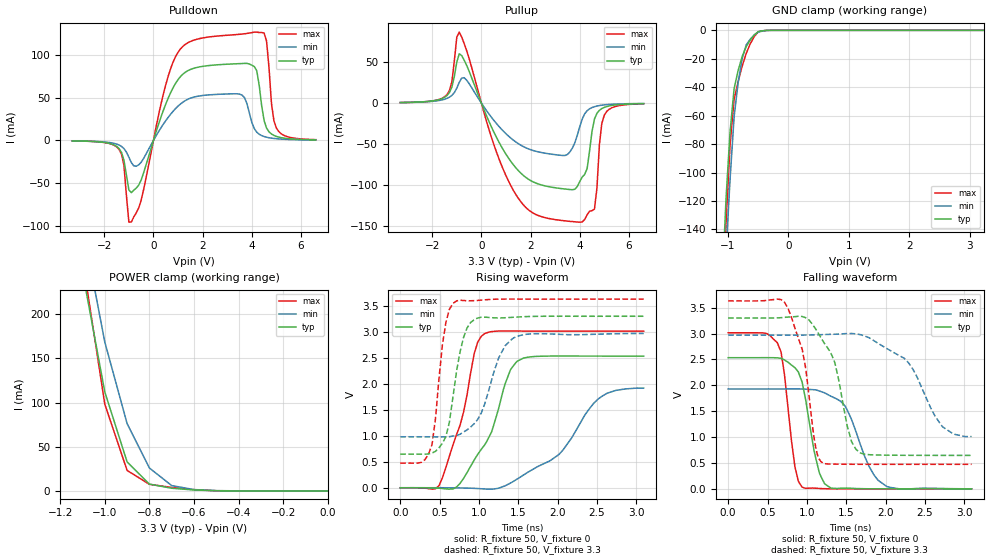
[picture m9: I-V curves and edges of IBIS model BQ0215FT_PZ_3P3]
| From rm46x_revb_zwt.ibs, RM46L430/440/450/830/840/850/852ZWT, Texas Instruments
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|   Model Cell BQ0215FT_PZ_3P3
|BQ0215FT_PZ_3P3
[Model]   BQ0215FT_PZ_3P3
Model_type   I/O
Polarity   Non-Inverting
Enable   Active-Low
Vinl =  1.15
Vinh =  1.55
Cref =  15.0001pF
Rref =  101.0000M
Vref =  0V
Vmeas =  1.65
C_comp   1.2p   1.2p   1.2p
[Model Spec]
Vinl   1.15   1.02   1.28
Vinh   1.55   1.45   1.65
[Temperature Range]   25   155   -40
[Voltage Range]   3.3   2.97   3.63
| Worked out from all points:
|   slope of the pulldown table from 0 to 0.495 V, typ, clamps not added: 11.7 ohm
|   slope of the pullup table from 0 to 0.495 V, typ, clamps not added: 14.3 ohm
|   GND clamp passes 1 mA (typ) near -0.50 V on its own axis
|   POWER clamp passes 1 mA (typ) near -0.59 V on its own axis
|   rising waveform, R_fixture 50, V_fixture 0: 20-80 % time 410ps typ, 692ps min, 296ps max; typ from 0 V to 2.53 V
|   rising waveform, R_fixture 50, V_fixture 3.3: 20-80 % time 174ps typ, 268ps min, 133ps max; typ from 0.647 V to 3.3 V
|   falling waveform, R_fixture 50, V_fixture 0: 20-80 % time 182ps typ, 302ps min, 138ps max; typ from 2.53 V to 0 V
|   falling waveform, R_fixture 50, V_fixture 3.3: 20-80 % time 278ps typ, 461ps min, 209ps max; typ from 3.3 V to 0.646 V
[POWER_clamp]
|   voltage   I(typ)   I(min)   I(max)
-3.3V     4.034A     4.621A     4.844A
-1.1V     248.3mA    300.9mA    262.9mA
-1.067V   202.9mA    256.8mA    208mA
-1.033V   157.5mA    212.7mA    153.2mA
-1V       112.1mA    168.6mA    98.31mA
-900mV    32.88mA    76.22mA    23.22mA
-800mV    7.705mA    25.94mA    7.475mA
-700mV    3.033mA    6.038mA    3.991mA
-600mV    1.087mA    1.528mA    1.425mA
-500mV    187uA      368.9uA    203.4uA
0V        579.1pA    13.17nA    479.4pA
[Pulldown]
|   voltage   I(typ)   I(min)   I(max)
-3.3V     -583.8uA   -509.7uA   -562.9uA
-1.4V     -9.427mA   -5.344mA   -10.39mA
-1.2V     -23.28mA   -9.543mA   -29.38mA
-1V       -58.07mA   -19.65mA   -95.88mA
-900mV    -61.21mA   -25.99mA   -95.59mA
1V        71.34mA    40.23mA    103.4mA
3.5V      90.06mA    54.34mA    124.5mA
4.2V      81.77mA    9.741mA    127mA
4.6V      14.51mA    3.766mA    116.4mA
4.8V      7.515mA    2.688mA    43.16mA
5V        4.703mA    2.013mA    14.54mA
6.6V      667.2uA    491.6uA    918.8uA
[Pullup]
|   voltage   I(typ)   I(min)   I(max)
-3.3V     645.2uA    598.5uA    584.2uA
-1.4V     9.107mA    5.632mA    10.27mA
-900mV    59.97mA    25.19mA    86.39mA
600mV     -40.93mA   -24.45mA   -58.47mA
1.4V      -78.76mA   -47.33mA   -111.2mA
3.4V      -104.6mA   -63.8mA    -143.4mA
4V        -95.69mA   -28.77mA   -145mA
4.3V      -79.78mA   -9.339mA   -136mA
4.6V      -19.38mA   -4.395mA   -129mA
4.8V      -8.841mA   -3.032mA   -50.9mA
5V        -5.243mA   -2.22mA    -14.75mA
6.6V      -699.3uA   -541.6uA   -880.5uA
[GND_clamp]
|   voltage   I(typ)   I(min)   I(max)
-3.3V     -3.232A    -2.867A    -4.906A
-1.1V     -181.4mA   -214mA     -212mA
-1.033V   -118mA     -155.8mA   -134.9mA
-966.7mV  -71.18mA   -104.7mA   -80.42mA
-900mV    -40.99mA   -60.83mA   -48.65mA
-833.3mV  -28.23mA   -36.87mA   -36.01mA
-766.7mV  -18.41mA   -20mA      -25.23mA
-700mV    -11.54mA   -10.23mA   -16.3mA
-566.7mV  -3.309mA   -3.247mA   -4.437mA
-500mV    -880.1uA   -1.256mA   -1.015mA
-300mV    -1.832uA   -15.98uA   -900.8nA
3.233V    553.4pA    4.097uA    367.7pA
[Ramp]
| variable   typ   min   max
dV/dt_f   1.613268/0.2883466n   1.213022/0.4924881n   1.916193/0.2144453n
dV/dt_r   1.537386/0.417794n   1.174541/0.7163023n   1.826409/0.2991251n
R_load = 50
[Rising Waveform]
R_fixture = 50
V_fixture = 0
V_fixture_min = 0
V_fixture_max = 0
|   time   V(typ)   V(min)   V(max)
0s        -1.134uV   -4.139uV   -934.2nV
492ps     -9.176mV   409.8uV    39.5mV
716ps     14.01mV    -2.646mV   1.026V
804ps     179.4mV    -5.212mV   1.456V
940ps     533.9mV    -11.54mV   2.583V
1.072ns   823mV      -23.66mV   2.966V
1.488ns   2.437V     169.9mV    3.015V
2.016ns   2.534V     640.6mV    3.014V
2.516ns   2.533V     1.711V     3.014V
3.092ns   2.533V     1.917V     3.014V
[Rising Waveform]
R_fixture = 50
V_fixture = 3.3
V_fixture_min = 2.97
V_fixture_max = 3.63
|   time   V(typ)   V(min)   V(max)
0s        646.5mV    980.1mV    473.8mV
268ps     646mV      980.2mV    487.6mV
404ps     667.9mV    979.6mV    831.7mV
580ps     985.4mV    979.7mV    3.183V
716ps     2.248V     1.007V     3.596V
892ps     3.177V     1.164V     3.598V
1.028ns   3.281V     1.434V     3.61V
1.248ns   3.267V     2.488V     3.629V
1.444ns   3.281V     2.886V     3.631V
3.092ns   3.3V       2.968V     3.63V
[Falling Waveform]
R_fixture = 50
V_fixture = 0
V_fixture_min = 0
V_fixture_max = 0
|   time   V(typ)   V(min)   V(max)
0s        2.534V     1.93V      3.014V
624ps     2.53V      1.93V      2.825V
716ps     2.49V      1.93V      2.204V
848ps     2.341V     1.931V     428.5mV
940ps     2.06V      1.929V     31.58mV
1.16ns    301.6mV    1.889V     7.441mV
1.292ns   27.53mV    1.8V       939.6uV
1.488ns   14.75mV    1.593V     217.4uV
2.016ns   492.8uV    44.47mV    213.7uV
3.092ns   277.9uV    1.352mV    30.68uV
[Falling Waveform]
R_fixture = 50
V_fixture = 3.3
V_fixture_min = 2.97
V_fixture_max = 3.63
|   time   V(typ)   V(min)   V(max)
0s        3.3V       2.97V      3.63V
760ps     3.318V     2.97V      3.489V
940ps     3.329V     2.97V      2.699V
1.092ns   3.132V     2.973V     980.3mV
1.18ns    2.916V     2.978V     522.3mV
1.356ns   2.431V     2.987V     477.9mV
1.68ns    692.1mV    2.978V     474.4mV
2.292ns   647.8mV    2.433V     474mV
2.724ns   646.5mV    1.198V     474mV
3.092ns   646.4mV    1.01V      473.9mV
